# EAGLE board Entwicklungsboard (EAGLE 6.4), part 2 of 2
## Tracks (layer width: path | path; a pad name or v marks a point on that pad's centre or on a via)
1A  (via drill 0.6)
  Top 0.3: v-144.73,27.65 -143.53,26.45 -143.53,24.05 JP15.15
  Bottom 0.3: v-144.73,27.65 -149.73,27.65 -157.63,35.55 IC8.2
1B  (via drill 0.6)
  Top 0.3: v-132.63,35.65 -132.63,46.65 -131.03,48.25 IC9.2
  Bottom 0.3: v-132.63,35.65 -141.63,26.65 -150.43,26.65 -151.43,25.65 -151.43,22.95 -152.53,22.95 JP15.7
1Y
  Top 0.3: IC8.3 -155.03,35.65 -154.53,36.15 -154.53,41.55 -154.03,42.05 -154.03,51.05 -155.03,52.05 MOTOR1.1
1YB
  Top 0.3: IC9.3 -128.33,48.35 -127.13,49.55 -127.13,62.25 -126.43,62.95 -115.73,62.95 -115.73,61.05 MOTOR2.1
2A
  Top 0.3: IC8.7 -144.93,35.55 -145.73,34.75 -145.73,26.25 -146.13,25.85 -146.13,24.15 -144.93,22.95 JP15.13
2B
  Bottom 0.3: IC9.7 -118.33,48.25 -121.03,45.55 -137.83,45.55 -146.03,37.35 -158.13,37.35 -158.73,36.75 -158.73,26.65 -154.63,26.65 -153.93,25.95 -153.93,22.95 -155.03,22.95 JP15.5
2Y
  Top 0.3: IC8.6 -147.53,35.65 -148.93,37.05 -148.93,51.05 -149.93,52.05 MOTOR1.3
2YB
  Top 0.3: IC9.6 -120.73,48.35 -119.73,49.35 -119.73,59.95 -120.73,60.95 MOTOR2.3
3A
  Top 0.3: IC8.10 -144.93,43.15 -146.33,41.75 -146.33,28.25 -148.63,25.95 -148.63,24.05 -147.53,22.95 JP15.11
3B
  Bottom 0.3: IC9.10 -118.33,55.95 -120.63,58.25 -152.23,58.25 -161.93,48.55 -161.93,21.75 -158.73,21.75 -157.63,22.85 JP15.3
3Y
  Top 0.3: IC8.11 -147.43,43.25 -147.43,52.05 MOTOR1.4
3YB
  Top 0.3: IC9.11 -120.83,55.95 -123.33,58.45 -123.33,60.95 MOTOR2.4
4A
  Top 0.3: IC8.15 -157.63,43.15 -156.23,41.75 -156.23,30.75 -151.13,25.65 -151.13,24.05 -150.03,22.95 JP15.9
4B
  Bottom 0.3: IC9.15 -131.03,55.95 -132.73,57.65 -152.03,57.65 -161.33,48.35 -161.33,22.95 -160.23,22.95 JP15.1
4Y
  Top 0.3: IC8.14 -155.13,43.25 -156.33,44.45 -156.33,53.35 -155.63,54.05 -142.43,54.05 -142.43,52.15 MOTOR1.6
4YB
  Top 0.3: IC9.14 -128.43,55.95 -128.43,60.95 MOTOR2.6
+12
  Top 0.3: -45.63,-13.68 S1.3 | -45.63,-9.08 S1.6 -45.53,-10.18 | C2.+ -48.33,2.52 -43.33,-2.48 -39.63,-2.48 TP4.TP -39.53,-2.58 -39.53,-10.08 C3.1 -39.63,-10.18
  Top 0.813: -45.63,-9.08 -45.63,-13.68 | -39.63,-10.18 -45.53,-10.18
  Bottom 0.3: -25.63,-15.18 IC1.1 | -39.43,-10.18 C3.1
  Bottom 0.813: -25.63,-15.18 -30.63,-10.18 -39.43,-10.18
+12V  (via drill 0.6)
  Top 0.3: v-115.83,43.95 -115.73,44.05 -115.73,48.25 IC9.8 | SPI_INPUT.3 -155.53,-10.55 -155.53,3.05 v-153.53,5.05
  Bottom 0.3: -131.63,40.85 -125.93,40.85 -122.83,43.95 v-115.83,43.95 | -131.63,40.85 -137.13,40.85 -142.33,35.65 IC8.8 | v-153.53,5.05 -148.93,9.65 -135.93,9.65 -132.53,13.05 -132.53,34.65 -132.23,34.65 -131.63,35.25 -131.63,40.85
A
  Top 0.3: A1.TP 63.14,149.83 63.14,146.33 10.1 62.79,145.98 62.79,136.18 10.2 62.79,135.83 62.79,130.93 11.1 63.14,130.58 63.14,126.03 66.99,126.03 67.34,125.68 69.79,125.68 70.49,124.98 70.49,123.23 65.59,123.23 63.14,120.78 11.2 62.79,120.78 62.79,115.88 12.1 62.79,115.53 62.79,105.73 12.2 | 18.2 62.79,90.33 62.79,100.13 18.1 62.79,100.48 62.79,105.38 12.2 | TASTATUR1.8 64.89,105.73 63.14,105.73 12.2
B  (via drill 0.6)
  Top 0.3: 59.29,148.43 59.99,147.73 59.99,143.88 56.49,143.88 | 59.29,148.43 58.94,148.78 55.79,148.78 54.74,149.83 B1.TP | 56.49,143.88 54.39,145.98 13.1 | 14.2 54.04,120.78 54.04,130.58 14.1 54.04,130.93 52.99,130.93 v52.29,131.63 | v51.94,133.73 54.04,135.83 13.2 | v56.49,138.98 56.49,143.88 | 19.2 54.04,90.33 54.04,100.13 19.1 54.04,100.48 54.04,103.63 | 54.04,103.63 54.04,105.38 15.2 | 60.34,103.63 60.34,107.13 59.29,108.18 54.39,108.18 54.39,115.53 15.1 | 54.04,103.63 60.34,103.63 | 60.34,103.63 60.34,89.63 61.74,88.23 70.49,88.23 70.49,109.93 68.74,111.68 TASTATUR1.7 68.39,112.03 66.29,112.03 66.29,119.73 67.34,120.78 71.19,120.78 71.19,144.58 64.19,151.58 62.44,151.58 59.29,148.43
  Bottom 0.3: v52.29,131.63 52.29,133.38 v51.94,133.73 51.94,134.43 v56.49,138.98
C  (via drill 0.6)
  Top 0.3: RIGHT1.2 45.29,90.33 45.29,100.13 RIGHT1.1 45.29,100.48 45.29,105.38 17.2 45.29,105.73 45.64,106.08 v47.74,106.08 | C16.TP 45.29,149.83 45.29,146.33 LEFT1.1 44.94,145.98 v44.94,142.13 | 16.2 45.29,118.33 | 45.29,118.33 45.29,115.88 17.1 | 16.2 45.29,130.58 16.1 44.94,130.93 43.89,130.93 v43.19,131.63 | 16.2 | v42.84,133.73 44.94,135.83 LEFT1.2 | v59.64,117.98 59.29,118.33 45.29,118.33
  Bottom 0.3: v43.19,131.63 43.19,133.38 v42.84,133.73 42.84,140.03 v44.94,142.13 | TASTATUR1.6 68.39,114.48 64.89,117.98 v59.64,117.98 v47.74,106.08
CS  (via drill 0.6)
  Top 0.3: IC2.11 -134.83,17.55 -134.83,19.45 -139.23,19.45 -139.93,18.75 -139.93,18.15 -146.93,11.15 -146.93,7.25 -147.43,6.75 IC3.11 -147.53,6.65 -147.53,5.55 v-148.03,5.05
  Bottom 0.3: SPI_INPUT.8 -156.93,0.75 -153.63,0.75 -151.03,3.35 -151.03,5.05 v-148.03,5.05
D
  Top 0.3: 36.19,128.83 36.19,130.58 F1.1 | 36.19,128.83 36.19,120.78 F1.2 | 29.19,133.38 33.74,133.38 36.19,135.83 CANCEL1.2 | 29.19,133.38 27.09,131.28 27.09,128.83 | 36.19,128.83 27.09,128.83 | 36.19,98.38 36.19,100.13 ENTER1.1 | 36.19,98.38 36.19,90.33 ENTER1.2 | 28.84,102.58 27.09,100.83 27.09,98.38 36.19,98.38 | 28.84,102.58 29.19,102.93 33.74,102.93 36.19,105.38 F3.2 | 28.84,108.18 36.19,115.53 F3.1 | 28.84,102.58 28.84,108.18 | 27.09,128.83 27.09,108.18 28.84,108.18 | 36.54,148.08 36.54,146.33 CANCEL1.1 | 36.54,148.08 36.54,149.83 D3.TP 36.89,150.18 38.99,152.28 66.99,152.28 69.79,149.48 73.24,145.67 73.24,120.78 72.89,120.43 72.24,120.43 68.74,116.93 TASTATUR1.5 | 29.19,133.38 29.19,144.23 28.49,144.23 27.09,145.63 27.09,148.08 36.54,148.08
DATA+
  Top 0.3: R52.1 59.36,-15.02 59.36,-12.62 64.16,-12.62 X1.3
DATA-  (via drill 0.6)
  Top 0.3: v60.86,-10.82 59.96,-10.82 59.36,-10.22 R53.1 | v61.76,-13.82 62.06,-13.52 64.16,-13.52 X1.2
  Bottom 0.3: v60.86,-10.82 61.76,-11.72 v61.76,-13.82
E  (via drill 0.6)
  Top 0.3: E1.TP 29.19,145.98 31.64,145.98 CANCEL1.3 31.99,145.98 34.09,143.88 40.74,143.88 | 40.74,143.88 40.74,145.98 LEFT1.3 | 40.74,143.88 40.74,141.08 | 40.74,141.08 40.74,137.93 | 40.74,137.93 40.74,136.18 LEFT1.4 | 40.74,137.93 33.74,137.93 31.99,136.18 CANCEL1.4 | 10.3 58.24,146.33 56.49,148.08 51.59,148.08 49.84,146.33 13.3 49.49,145.98 49.49,141.08 | v62.09,125.68 62.09,128.83 61.74,128.83 59.99,130.58 59.99,135.83 58.59,135.83 10.4 58.24,136.18 56.49,137.93 51.59,137.93 49.84,136.18 13.4 49.49,136.18 49.49,141.08 | 49.49,141.08 40.74,141.08
  Bottom 0.3: v62.09,125.68 62.09,119.73 68.39,119.73 TASTATUR1.4
F  (via drill 0.6)
  Top 0.3: 58.59,124.63 58.59,130.58 11.3 58.24,130.93 56.49,132.68 47.74,132.68 | 58.59,124.63 58.59,120.78 11.4 | v64.89,124.98 64.54,124.63 58.59,124.63 | 14.4 49.49,120.78 49.49,130.58 14.3 49.49,130.93 47.74,132.68 | F2.TP 29.19,130.93 31.64,130.93 F1.3 31.99,130.93 33.74,132.68 38.99,132.68 | 40.74,120.78 40.74,130.58 16.3 40.74,130.93 38.99,132.68 | 40.74,120.78 38.64,118.68 34.09,118.68 31.99,120.78 F1.4 | 40.74,120.78 16.4 | 38.99,132.68 47.74,132.68
  Bottom 0.3: v64.89,124.98 64.89,122.18 68.39,122.18 TASTATUR1.3
G
  Top 0.3: TASTATUR1.2 68.39,124.28 68.04,123.93 63.14,123.93 60.69,121.48 60.69,115.88 58.59,115.88 12.3 58.24,115.88 56.49,117.63 51.59,117.63 49.84,115.88 15.3 49.49,115.53 47.39,113.43 40.74,113.43 | 12.4 58.24,105.73 56.49,107.48 51.59,107.48 49.84,105.73 15.4 49.49,105.73 47.74,107.48 40.74,107.48 | G1.TP 29.19,115.53 31.64,115.53 F3.3 31.99,115.88 33.74,117.63 38.99,117.63 40.74,115.88 17.3 40.74,115.53 40.74,113.43 | 40.74,113.43 40.74,107.48 | 40.74,107.48 40.74,105.73 17.4 | 40.74,107.48 33.74,107.48 31.99,105.73 F3.4
GND
  Top 0.8: C5.1 -8.63,39.42 -8.13,38.92 -8.13,36.12 -6.93,34.92 -6.93,21.22 -9.03,19.12 SG1.- | -0.33,38.02 -1.63,38.02 -1.63,48.52 U1.12 -2.83,49.92 -6.53,53.62 -6.53,63.62 -7.73,64.82 U1.31 | -0.33,38.02 2.37,38.02 2.77,38.42 2.77,38.92 3.27,39.42 C6.2 | -0.33,38.02 -0.33,32.12 0.67,32.12 7.27,25.52 11.27,25.52 JP3.3 11.67,25.32 20.47,16.52 20.47,4.32 19.07,2.92 IR1.GND 18.87,2.52 13.57,-2.78 13.57,-15.08 11.37,-17.28 C8.- 11.27,-17.68 -2.63,-17.68 C7.2 | JP19.2 20.17,85.22 19.07,86.32 19.07,86.52 -3.13,108.72 -7.43,108.72 R22.2 -7.83,109.02 -10.53,109.02 -10.93,109.42 -21.43,109.42 -21.43,109.22 R23.2 -21.83,108.92 -31.83,108.92 R20.2 -32.23,108.72 -35.13,108.72 -35.13,81.72 R10.2 -35.43,81.42 -38.23,81.42 | C9.- -49.23,41.92 -49.23,34.82 -50.93,33.12 C1.- -50.83,32.72 -49.73,31.62 -49.73,19.22 -48.63,18.12 C10.1 -48.43,17.82 -48.43,10.22 C2.- -48.13,9.92 -37.53,-0.68 -37.53,-15.78 -39.43,-17.68 C3.2 | ICSP.3 -40.73,58.52 -39.63,58.52 -39.63,59.32 -38.33,60.62 -38.33,73.62 C4.- -38.23,74.02 -38.23,81.42 | -50.93,83.82 -50.93,83.62 S2.4 | -38.23,81.42 -40.83,81.42 -40.83,83.52 S2.3 -41.23,83.62 -50.53,83.62 S2.4 | TP6.TP -52.13,87.62 -51.13,86.62 -51.13,84.12 S2.4
  Bottom 0.8: SG1.- -9.03,19.12 -2.73,25.42 11.27,25.42 JP3.3 | GND.1 -43.33,-20.18 -41.93,-20.18 -39.53,-17.78 C3.2 -39.33,-17.38 -23.03,-17.38 | -23.03,-17.38 -23.03,-15.28 IC1.2 | -23.03,-17.38 -22.73,-17.58 -22.63,-17.68 -2.73,-17.68 C7.2 | C9.- -49.13,42.02 -46.63,44.52 -46.63,58.42 -40.83,58.42 ICSP.3
GNDCOM
  Top 0.3: 47.91,20.93 47.91,27.93 C15.1 | 46.76,20.93 45.11,20.93 44.41,20.23 | 46.76,20.93 47.91,20.93 | 62.36,-11.12 61.46,-12.02 48.86,-12.02 43.16,-17.72 JP16.1 | 62.66,-11.12 64.16,-11.12 X1.5 62.66,-11.12 | 62.66,-11.12 62.36,-11.12 | 46.76,20.98 46.76,20.93 | 49.26,15.68 47.26,13.68 45.86,13.68 45.86,2.48 IC10.7 | 49.26,15.68 49.26,20.98 47.96,20.98 47.91,20.93 | IC10.26 48.46,-4.82 47.86,-4.82 IC10.25 47.86,-4.92 47.86,-6.02 | 45.06,-5.92 45.26,-5.72 45.26,-4.92 IC10.21 | 45.06,-5.92 44.96,-6.02 43.26,-6.02 43.26,-4.92 IC10.18 | 47.86,-6.02 45.16,-6.02 45.06,-5.92 | 58.56,-5.82 59.26,-5.12 C11.2 59.26,-5.02 60.56,-3.72 67.06,-3.72 67.16,-3.62 67.16,8.08 66.16,9.08 55.86,9.08 49.26,15.68 | 58.56,-5.82 58.16,-6.22 48.06,-6.22 47.86,-6.02 | 58.56,-5.82 62.16,-9.42 62.26,-9.42 62.26,-11.02 62.36,-11.12
  Bottom 0.3: IC11.15 48.26,46.83 53.16,41.93 53.16,36.33 54.21,35.28 X2.5 54.21,34.93 54.21,34.23 48.26,28.28 C15.1 48.26,27.93 49.31,26.88
  pour Bottom (isolate 0.406): 74.78,61.01 74.78,-22.81 30.33,-22.81 30.33,61.01
GNDI2C
  Top 0.3: -154.02,130.4 -154.02,128.65 -153.32,127.95 -153.32,127.25 U$1.4 | -154.02,130.4 -154.02,131.8 -154.37,132.15 U$1.6 | -154.02,130.4 -162.42,130.4 -162.42,143.35 R65.E
  pour Bottom (isolate 0.406): -172.87,153.72 -80.16,153.72 -80.16,80.06 -172.87,80.06
GNDSPI  (via drill 0.6)
  Top 0.3: LED17.13 -106.83,-1.05 | -106.83,-1.05 LED17.14 -106.93,-2.45 -114.83,-2.45 -114.83,-10.85 -117.73,-13.75 -117.73,-14.35 -118.73,-15.35 -127.13,-15.35 -127.13,-16.35 IC5.8 -127.23,-16.55 -129.93,-19.25 -156.33,-19.25 -156.33,-13.95 SPI_INPUT.2 -156.23,-13.85 -154.93,-12.55 -154.93,-6.95 -149.03,-1.05 -149.03,6.25 -148.73,6.55 IC3.10 -148.73,6.75 -148.23,7.25 -148.23,12.15 -146.23,14.15 -146.23,16.25 IC3.17 -146.13,16.25 IC3.16 -144.83,16.25 -143.73,16.25 IC3.15 -143.63,16.35 -143.63,20.05 -141.23,20.05 | -92.73,-1.05 -92.73,6.45 -91.63,7.55 LED17.9 | -92.73,-1.05 -92.73,-3.95 -91.63,-5.05 LED17.4 | -92.73,-1.05 -106.83,-1.05 | LED18.13 LED18.14 | IC4.8 -71.33,3.95 -78.83,11.45 -78.83,19.05 IC7.8 | LED18.4 -92.73,23.95 -92.73,34.35 -91.63,35.45 LED18.9 | IC8.13 -152.53,43.25 -150.03,43.25 IC8.12 | MOTOR1.2 -152.53,52.05 -152.53,43.35 IC8.13 | IC8.4 -152.53,35.65 -152.53,43.15 IC8.13 | -124.63,48.35 -123.43,48.35 IC9.5 -123.23,48.25 -123.23,45.75 -119.53,42.05 IC6.8 | -124.63,48.35 -125.83,48.35 IC9.4 | -124.63,55.95 -123.43,55.95 IC9.12 | -124.63,55.95 -125.83,55.95 IC9.13 -125.83,56.05 -125.83,60.95 MOTOR2.5 | -124.63,55.95 -124.63,48.35 | -141.23,20.05 -134.63,20.05 -134.03,19.45 -134.03,18.05 -133.53,17.55 IC2.10 | v-142.03,27.65 -141.23,26.85 -141.23,20.05
  Bottom 0.3: -88.63,19.85 -79.63,19.85 -78.93,19.15 IC7.8 | -88.63,19.85 LED18.4 -91.73,22.85 -94.03,25.15 -106.43,25.15 LED18.14 | LED17.9 -91.53,7.65 -88.73,10.45 -88.73,19.75 -88.63,19.85 | IC8.4 -152.53,35.65 -150.03,35.65 IC8.5 -149.93,35.55 v-142.03,27.65 | MOTOR1.2 -152.53,52.15 -150.63,54.05 -146.83,54.05 -144.93,52.15 MOTOR1.5 -144.83,52.05 -142.83,50.05 -127.63,50.05 -125.93,48.35 IC9.4 | MOTOR2.2 -118.33,61.05 -120.23,62.95 -123.93,62.95 -125.83,61.05 MOTOR2.5
H  (via drill 0.6)
  Top 0.3: 19.4 49.49,90.33 49.49,100.13 19.3 | H1.TP 29.19,100.48 31.64,100.48 ENTER1.3 31.99,100.48 33.74,102.23 38.99,102.23 40.74,100.48 RIGHT1.3 40.74,100.13 40.74,90.33 RIGHT1.4 40.74,89.98 38.99,88.23 | 38.99,88.23 33.74,88.23 31.99,89.98 ENTER1.4 | 38.99,88.23 47.74,88.23 49.49,89.98 19.4 | 18.3 58.59,100.13 58.59,90.33 18.4 58.59,89.98 60.34,88.23 | v72.59,119.38 72.24,110.54 72.24,88.45 71.32,87.53 61.04,87.53 60.34,88.23 | 60.34,88.23 51.59,88.23 49.84,89.98 19.4
  Bottom 0.3: v72.59,119.38 72.59,122.88 68.74,126.73 TASTATUR1.1
MCLR
  Top 0.3: D2.C -44.53,49.62 -40.83,53.32 ICSP.1
  Bottom 0.3: U1.1 -30.63,49.62 -34.33,53.32 -40.73,53.32 ICSP.1
N$1
  Top 0.3: C5.2 -6.73,39.42 -4.03,42.12 -4.03,44.42 Q1.1
  Bottom 0.3: U1.13 -0.23,49.52 -3.93,45.82 -3.93,44.52 Q1.1
N$2
  Top 0.3: R2.1 -20.43,138.72 -20.43,134.72 JP5.8
N$3
  Top 0.3: C6.1 1.37,39.42 1.17,39.62 1.17,44.42 Q1.2 1.17,44.62 1.17,48.32 2.37,49.52 U1.14
N$4
  Top 0.3: JP5.7 R3.1
N$5
  Top 0.3: R13.1 -42.33,113.12 -38.33,113.12 JP10.8
N$6
  Top 0.3: JP10.7 R14.1
N$7
  Top 0.3: R15.1 -42.33,118.22 -38.33,118.22 JP10.6
N$8
  Top 0.3: R16.1 -42.33,120.72 -38.33,120.72 JP10.5
N$9
  Top 0.3: R17.1 -42.33,123.32 -38.33,123.32 JP10.4
N$10
  Top 0.3: R18.1 -42.33,125.82 -38.33,125.82 JP10.3
N$11
  Top 0.3: JP10.2 R19.1
N$12
  Top 0.3: R21.1 -42.33,130.92 -38.33,130.92 JP10.1
N$13
  Top 0.3: R13.2 -44.33,113.02 -47.93,109.42 -47.93,97.02 -49.63,95.32 LED9.K
N$14
  Top 0.3: R15.2 -44.33,118.12 -49.63,112.82 -49.63,110.62 LED11.K
N$15
  Top 0.3: R16.2 -44.33,120.62 -49.63,120.62 -49.63,118.22 LED12.K
N$16
  Top 0.3: R17.2 -44.33,123.32 -49.63,123.32 -49.63,125.72 LED13.K
N$17
  Top 0.3: R21.2 -44.33,130.92 -47.93,134.52 -47.93,146.92 -49.63,148.62 LED16.K
N$18
  Top 0.3: R18.2 -44.33,125.82 -49.63,131.12 -49.63,133.32 LED14.K
N$19
  Top 0.3: R14.2 -44.33,115.62 -48.53,111.42 -48.53,104.02 -49.63,102.92 LED10.K
N$20
  Top 0.3: R19.2 -44.33,128.32 -48.53,132.52 -48.53,139.92 -49.63,141.02 LED15.K
N$21
  Top 0.3: R4.1 -15.33,138.72 -15.33,134.72 JP5.6
N$22
  Top 0.3: R6.1 -12.83,138.72 -12.83,134.72 JP5.5
N$23
  Top 0.3: R7.1 -10.23,138.72 -10.23,134.72 JP5.4
N$24
  Top 0.3: R9.1 -7.73,138.72 -7.73,134.72 JP5.3
N$25
  Top 0.3: JP5.2 R11.1
N$26
  Top 0.3: R12.1 -2.63,138.72 -2.63,134.72 JP5.1
N$27
  Top 0.3: R2.2 -20.53,140.72 -27.33,147.52 -38.23,147.52 -38.23,148.62 LED1.K
N$28
  Top 0.3: R4.2 -15.43,140.72 -22.93,148.22 -22.93,148.62 LED3.K
N$29
  Top 0.3: R6.2 -12.93,140.72 -15.33,143.12 -15.33,148.62 LED4.K
N$30
  Top 0.3: R7.2 -10.23,140.72 -7.83,143.12 -7.83,148.62 LED5.K
N$31
  Top 0.3: R12.2 -2.63,140.72 4.17,147.52 15.07,147.52 15.07,148.62 LED8.K
N$32
  Top 0.3: R3.2 -17.93,140.72 -25.83,148.62 -30.63,148.62 LED2.K
N$33
  Top 0.3: R9.2 -7.73,140.72 -0.23,148.22 -0.23,148.62 LED6.K
N$34
  Top 0.3: R11.2 -5.23,140.72 2.67,148.62 7.47,148.62 LED7.K
N$35
  Top 0.3: IC11.14 47.91,44.38 46.16,42.63 46.16,40.88 54.21,40.88 X2.3
N$36
  Top 0.3: IC11.13 48.26,42.28 49.31,43.33 54.21,43.33 X2.2
N$37
  Bottom 0.3: IC11.2 40.56,47.18 42.31,48.93 42.31,51.38 40.56,53.13 C14.2
N$38
  Bottom 0.3: IC11.6 40.56,36.68 42.31,34.93 42.31,30.03 40.56,28.28 C15.2
N$39
  Top 0.3: IC11.3 40.21,44.73 38.11,46.83 34.26,46.83 C12.2
N$40
  Top 0.3: IC11.1 40.21,49.63 35.31,54.53 34.26,54.53 C12.1
N$41
  Top 0.3: IC11.4 40.21,42.28 39.51,42.98 34.26,42.98 C13.1
N$42
  Top 0.3: IC11.5 40.21,39.13 36.71,35.63 34.26,35.63 C13.2
N$43  (via drill 0.6)
  Top 0.3: v47.46,-2.22 45.86,-2.22 45.86,-4.82 IC10.22 | v55.16,5.48 57.26,7.58 R56.1
  Bottom 0.3: v55.16,5.48 v47.46,-2.22
N$44  (via drill 0.6)
  Top 0.3: v51.96,-0.62 49.36,-3.22 46.56,-3.22 46.56,-4.82 IC10.23 | v56.16,12.58 56.16,13.98 57.26,13.98 R55.1
  Bottom 0.3: v51.96,-0.62 56.16,3.58 v56.16,12.58
N$45
  Top 0.3: 59.36,17.68 LED19.K 59.26,17.58 59.26,14.08 R55.2
N$46
  Top 0.3: 63.26,7.48 LED20.K 63.16,7.58 59.26,7.58 R56.2
N$47
  Top 0.3: IC10.17 42.66,-4.82 42.66,-3.22 34.46,-3.22 34.16,-2.92 34.16,0.78 47.46,0.78 47.86,0.38 53.06,0.38 57.26,-3.82 57.26,-5.02 C11.1
N$48
  Top 0.3: R22.1 -7.83,107.02 -8.03,106.82 -8.03,104.12 INT1.4 -8.03,104.02 -8.03,94.12 INT1.3
N$49
  Top 0.3: R52.2 57.26,-15.32 52.76,-19.82 41.36,-19.82 41.36,-4.92 IC10.15
N$50
  Top 0.3: IC12.4 -97.67,127.25 -93.47,127.25 -93.47,128.65 -91.37,130.75 -82.27,130.75 -82.27,104.5 -85.07,101.7 KEYBOARD.1
N$51
  Top 0.3: IC12.5 -98.02,124.45 -110.62,111.85 -113.77,111.85 -113.77,107.65 -112.72,106.6 -87.17,106.6 -87.17,106.25 -85.42,104.5 KEYBOARD.2
N$52  (via drill 0.6)
  Top 0.3: 43.71,29.33 48.61,29.33 50.36,27.58 50.36,19.18 JP18.3 | v49.86,13.68 49.86,2.48 IC10.1
  Bottom 0.3: 50.36,18.88 JP18.3 50.26,18.78 50.26,14.08 v49.86,13.68
N$53  (via drill 0.6)
  Top 0.3: v-94.52,122 -92.07,119.55 -92.07,113.6 -85.42,106.95 KEYBOARD.3
  Bottom 0.3: v-94.52,122 -97.67,122 IC12.6
N$54
  Bottom 0.3: IC12.7 -97.67,119.2 -96.62,119.2 -87.17,109.75 -86.82,109.75 -86.47,109.4 -85.42,109.4 KEYBOARD.4
N$55
  Top 0.3: R53.2 57.26,-9.92 41.96,-9.92 41.96,-4.92 IC10.16
N$56
  Bottom 0.3: IC11.11 45.81,34.58 45.81,19.18 JP18.1
N$57
  Top 0.3: JP6.1 R8.2
N$58  (via drill 0.6)
  Top 0.3: v47.16,12.68 47.16,2.48 IC10.5 | v46.86,14.68 42.46,19.08 41.76,19.08 JP17.3
  Bottom 0.3: 43.76,17.08 41.76,19.08 JP17.3 | v47.16,12.68 46.86,12.98 v46.86,14.68
N$59
  Top 0.3: IC11.12 47.91,39.13 41.96,33.18 36.86,33.18 | 36.86,33.18 36.71,33.18 | 36.86,33.18 36.86,19.18 JP17.1 | 36.86,33.28 36.86,33.18
N$60
  Top 0.3: IC12.9 -90.32,116.75 -85.42,111.85 KEYBOARD.5
N$61
  Top 0.3: IC12.10 -90.32,119.2 -85.42,114.3 KEYBOARD.6
N$62
  Top 0.3: IC12.11 -90.32,121.65 -82.97,121.65 -82.97,119.2 -85.07,117.1 KEYBOARD.7
N$63
  Top 0.3: IC12.12 -90.32,124.45 -92.07,122.7 -92.07,121.3 -91.37,120.6 -85.42,120.6 -85.42,119.55 KEYBOARD.8
N$64
  Top 0.3: IC10.19 43.96,-4.82 43.96,-2.22 35.46,-2.22 R54.2
N$65
  Bottom 0.3: IC4.7 -71.23,1.25 -68.93,-1.05 -68.93,-19.25 -146.33,-19.25 -148.83,-16.75 -148.83,-13.95 -149.93,-13.95 JP13.15
N$66
  Top 0.3: R5.2 -28.03,70.92 -28.03,85.12 JP6.2
N$67
  Bottom 0.3: IC4.1 -71.33,-13.95 -72.43,-15.05 -146.33,-15.05 -147.43,-13.95 JP13.13
N$68  (via drill 0.6)
  Top 0.3: v-143.73,-18.25 -143.73,-15.15 -144.93,-13.95 JP13.11
  Bottom 0.3: v-143.73,-18.25 -69.53,-18.25 -69.53,-13.15 -71.23,-11.45 IC4.2
N$69  (via drill 0.6)
  Top 0.3: v-81.33,-10.85 -81.33,-7.75 -77.83,-7.75 -71.33,-1.25 IC4.6
  Bottom 0.3: v-81.33,-10.85 -81.83,-11.35 -117.33,-11.35 -118.43,-10.25 -137.53,-10.25 -140.03,-12.75 -141.23,-12.75 -142.33,-13.85 JP13.9
N$70
  Bottom 0.3: IC5.7 -127.23,-13.85 -128.33,-12.75 -138.73,-12.75 -139.83,-13.85 JP13.7
N$71  (via drill 0.6)
  Top 0.3: v-136.83,-2.75 -137.23,-3.15 -137.23,-13.85 JP13.5
  Bottom 0.3: v-136.83,-2.75 -135.83,-1.75 -130.23,-1.75 -127.23,1.25 IC5.1
N$72  (via drill 0.6)
  Top 0.3: v-132.23,-2.75 -133.83,-4.35 -133.83,-9.15 -134.73,-10.05 -134.73,-13.85 JP13.3
  Bottom 0.3: v-132.23,-2.75 -128.73,-2.75 -127.23,-1.25 IC5.2
N$73  (via drill 0.6)
  Top 0.3: v-130.73,-11.75 -132.23,-13.25 JP13.1
  Bottom 0.3: v-130.73,-11.75 -127.53,-11.75 -127.23,-11.45 IC5.6
N$74  (via drill 0.6)
  Top 0.3: v-134.83,-4.75 -134.83,-3.95 -130.93,-0.05 -130.93,7.95 IC2.21 | v-145.63,-10.45 -148.83,-13.65 -148.83,-15.35 -149.93,-16.45 JP13.16
  Bottom 0.3: v-134.83,-4.75 -140.53,-10.45 v-145.63,-10.45
N$75  (via drill 0.6)
  Top 0.3: v-132.83,-4.75 -130.23,-2.15 -130.23,7.45 -129.73,7.95 IC2.22 | v-144.03,-11.45 -146.33,-13.75 -146.33,-15.35 -147.43,-16.45 JP13.14
  Bottom 0.3: v-132.83,-4.75 -139.53,-11.45 v-144.03,-11.45
N$76
  Top 0.3: R25.2 -87.53,-10.15 -91.53,-10.15 LED17.2
N$77  (via drill 0.6)
  Top 0.3: v-112.03,-3.45 -112.03,-4.15 -112.83,-4.95 R24.1
  Bottom 0.3: v-112.03,-3.45 -111.73,-3.75 -78.93,-3.75 IC4.12
N$78  (via drill 0.6)
  Top 0.3: v-90.33,-6.25 -111.63,-6.25 -112.03,-6.65 -112.03,-6.75 -112.83,-7.55 R37.1
  Bottom 0.3: v-90.33,-6.25 -78.93,-6.25 IC4.13
N$79  (via drill 0.6)
  Top 0.3: v-84.23,-8.85 -84.23,-10.05 -85.53,-10.05 R25.1 | v-82.23,-7.25 -80.63,-5.65 -80.63,-0.45 -78.93,1.25 IC4.10
  Bottom 0.3: v-84.23,-8.85 -82.63,-7.25 v-82.23,-7.25
N$80
  Top 0.3: R38.1 -85.53,-7.55 -83.83,-5.85 -83.83,1.15 -80.03,4.95 -77.13,4.95 -77.13,0.55 -78.83,-1.15 IC4.11
N$81
  Top 0.3: R39.1 -85.53,-12.65 -83.23,-10.35 -83.23,-0.45 -78.93,3.85 IC4.9
N$82
  Top 0.3: R26.1 -112.83,-12.65 -112.03,-13.45 -112.03,-13.55 -108.23,-17.35 -80.63,-17.35 -80.63,-13.15 -78.93,-11.45 IC4.15
N$83  (via drill 0.6)
  Top 0.3: v-107.73,-8.95 -111.83,-8.95 -112.03,-9.15 -112.03,-9.25 -112.83,-10.05 R40.1
  Bottom 0.3: v-107.73,-8.95 -107.63,-9.05 -85.43,-9.05 -84.63,-9.85 -79.93,-9.85 -78.93,-8.85 IC4.14
N$84  (via drill 0.6)
  Top 0.3: v-115.83,-2.55 -115.83,2.15 -112.93,5.05 R41.1
  Bottom 0.3: v-115.83,-2.55 -119.53,-6.25 IC5.13
N$85
  Top 0.3: R27.1 -112.93,7.65 -116.83,3.75 -116.83,-10.85 -118.43,-12.45 -121.33,-12.45 -121.33,-10.65 IC5.12
N$86
  Top 0.3: R42.1 -85.63,5.15 -86.33,5.85 -86.33,6.05 -89.23,8.95 -117.73,8.95 -117.73,-9.55 -119.53,-11.35 IC5.11
N$87  (via drill 0.6)
  Top 0.3: v-84.83,-4.75 -84.43,-4.35 -84.43,-1.05 -85.53,0.05 R28.1
  Bottom 0.3: v-84.83,-4.75 -84.43,-5.15 -77.83,-5.15 -77.13,-5.85 -77.13,-12.65 -89.83,-12.65 -91.13,-13.95 -119.53,-13.95 IC5.10
N$88
  Top 0.3: R43.1 -85.63,-2.55 -86.33,-3.25 -86.33,-3.65 -90.43,-7.75 -90.43,-8.15 -91.33,-9.05 -105.63,-9.05 -105.63,-10.65 -106.43,-11.45 -114.63,-11.45 -114.63,-12.05 -119.03,-16.45 IC5.9
N$89  (via drill 0.6)
  Top 0.3: v-114.83,0.65 -112.93,2.55 R29.1
  Bottom 0.3: v-114.83,0.65 -116.63,-1.15 -119.53,-1.15 IC5.15
N$90  (via drill 0.6)
  Top 0.3: v-84.03,2.55 -85.53,2.55 R44.1
  Bottom 0.3: v-84.03,2.55 -87.83,-1.25 -115.93,-1.25 -118.43,-3.75 IC5.14
N$91
  Top 0.3: R37.2 -110.93,-7.65 -106.83,-7.65 LED17.16
N$92
  Top 0.3: R24.2 -110.93,-5.05 -106.83,-5.05 LED17.15
N$93  (via drill 0.6)
  Top 0.3: v-88.93,-7.65 -87.53,-7.65 R38.2
  Bottom 0.3: v-88.93,-7.65 -91.53,-7.65 LED17.3
N$94
  Top 0.3: R39.2 -91.53,-12.65 -91.53,-12.75 LED17.1
N$95
  Top 0.3: R26.2 -106.83,-12.65 LED17.18
N$96
  Top 0.3: R40.2 -110.93,-10.15 -106.83,-10.15 LED17.17
N$97
  Top 0.3: R41.2 -110.93,5.15 -106.83,5.15 LED17.11
N$98
  Top 0.3: R27.2 -110.93,7.75 -106.83,7.75 LED17.10
N$99
  Top 0.3: R42.2 -87.53,5.05 -91.53,5.05 LED17.8
N$100
  Top 0.3: R28.2 -91.53,0.05 -91.53,-0.05 LED17.6
N$101
  Top 0.3: R43.2 -87.53,-2.55 -91.53,-2.55 LED17.5
N$102
  Top 0.3: R29.2 -110.93,2.65 -106.83,2.65 LED17.12
N$103
  Top 0.3: R44.2 -87.53,2.55 -91.53,2.55 LED17.7
N$104  (via drill 0.6)
  Top 0.3: v-130.63,-16.45 -130.63,-13.05 -128.93,-11.35 -128.93,7.45 -128.43,7.95 IC2.23
  Bottom 0.3: v-130.63,-16.45 -131.83,-17.65 -142.93,-17.65 -144.03,-16.55 -144.93,-16.55 JP13.12
N$105  (via drill 0.6)
  Top 0.3: v-127.63,6.25 -127.63,7.55 -127.23,7.95 IC2.24 | v-131.93,5.25 -141.23,-4.05 -141.23,-15.35 -142.33,-16.45 JP13.10
  Bottom 0.3: v-127.63,6.25 -128.63,5.25 v-131.93,5.25
N$106  (via drill 0.6)
  Top 0.3: v-126.03,6.25 -126.03,7.85 -125.93,7.95 IC2.25 | v-131.93,3.85 -138.73,-2.95 -138.73,-15.35 -139.83,-16.45 JP13.8
  Bottom 0.3: v-126.03,6.25 -128.43,3.85 v-131.93,3.85
N$107  (via drill 0.6)
  Top 0.3: IC2.26 -124.83,7.75 v-124.83,4.65 | v-131.93,2.45 -135.83,-1.45 -135.83,-13.35 -136.13,-13.65 -136.13,-15.35 -137.23,-16.45 JP13.6
  Bottom 0.3: v-124.83,4.65 -127.03,2.45 v-131.93,2.45
N$108  (via drill 0.6)
  Top 0.3: v-123.83,-5.15 -123.83,7.55 -123.43,7.95 IC2.27 | v-131.63,-7.75 -133.63,-9.75 -133.63,-15.35 -134.73,-16.45 JP13.4
  Bottom 0.3: v-123.83,-5.15 -126.43,-7.75 v-131.63,-7.75
N$109
  Top 0.3: JP13.2 -132.23,-17.45 -130.23,-17.45 -129.63,-16.85 -129.63,-12.85 -126.43,-12.85 -122.53,-8.95 -122.53,7.55 -122.13,7.95 IC2.28
N$110  (via drill 0.6)
  Top 0.3: v-116.83,49.95 -116.83,47.55 -117.83,46.55 -117.83,45.55 -117.73,45.45 -117.73,41.25 -119.53,39.45 IC6.7
  Bottom 0.3: v-116.83,49.95 -110.93,55.85 -108.13,55.85 JP14.15
N$111  (via drill 0.6)
  Top 0.3: v-114.73,24.45 -113.73,25.45 -113.73,29.35 -113.93,29.55 -113.93,45.95 -106.73,53.15 -106.73,54.75 -105.63,55.85 JP14.13
  Bottom 0.3: v-114.73,24.45 -119.33,24.45 -119.53,24.25 IC6.1
N$112  (via drill 0.6)
  Top 0.3: v-114.73,27.05 -114.73,47.05 -110.63,51.15 -110.63,55.85 -108.83,57.65 -103.03,57.65 -103.03,55.95 JP14.11
  Bottom 0.3: v-114.73,27.05 -119.23,27.05 -119.53,26.75 IC6.2
N$113  (via drill 0.6)
  Top 0.3: v-103.83,43.95 -101.63,46.15 -101.63,54.75 -100.53,55.85 JP14.9
  Bottom 0.3: v-103.83,43.95 -112.53,43.95 -119.53,36.95 IC6.6
N$114
  Top 0.3: IC7.7 -78.93,21.65 -82.63,25.35 -82.63,44.05 -91.73,53.15 -91.73,53.85 -92.63,54.75 -97.93,54.75 -97.93,55.85 JP14.7
N$115
  Bottom 0.3: IC7.1 -78.93,36.95 -89.13,47.15 -89.13,54.75 -94.23,54.75 -95.33,55.85 JP14.5
N$116
  Top 0.3: IC7.2 -78.93,34.35 -81.43,36.85 -81.43,48.65 -89.83,57.05 -92.83,57.05 -92.83,55.95 JP14.3
N$117
  Top 0.3: IC7.6 -78.93,24.25 -82.03,27.35 -82.03,47.65 -90.23,55.85 JP14.1
N$118
  Top 0.3: R20.1 -31.83,107.02 -31.63,106.82 -31.63,104.12 INT2.3 -31.53,104.02 -31.53,94.12 INT2.4
N$119
  pour Bottom (isolate 0.61): 26.52,83.87 26.52,153.72 76.05,153.72 76.05,83.87
N$120
  pour Top (isolate 0.813): -56.03,154.99 22.71,154.99 22.71,-22.81 -56.03,-22.81
N$121
  Bottom 0.305: 43.93,0.34 43.98,0.39
N$122
  Top 0.3: JP2.1 -9.03,31.72 SG1.+
N$137
  Top 0.3: JP3.2 18.87,15.32 18.87,10.22 IR1.VO
N$150  (via drill 0.6)
  Top 0.3: v-150.83,17.95 -150.83,16.75 -151.23,16.35 IC3.21
  Bottom 0.3: v-150.83,17.95 -146.13,22.65 -146.13,24.25 -143.63,24.25 -142.43,25.45 JP15.16
N$151
  Top 0.3: JP15.14 -144.93,24.65 -143.73,23.45 -143.73,21.15 -149.03,21.15 -152.03,18.15 -152.03,16.85 -152.53,16.35 IC3.22
N$152  (via drill 0.6)
  Top 0.3: IC3.23 -153.33,16.75 v-153.33,17.95
  Bottom 0.3: v-153.33,17.95 -148.63,22.65 -148.63,25.45 JP15.12
N$153
  Top 0.3: IC3.24 -155.03,16.35 -154.63,16.75 -154.63,18.25 -151.13,21.75 -148.83,21.75 -148.83,23.45 -149.93,24.55 -149.93,25.45 JP15.10
N$154
  Top 0.3: IC3.25 -156.33,16.35 -155.83,16.85 -155.83,20.55 -153.73,22.65 -153.73,24.35 -152.63,25.45 JP15.8
N$155
  Top 0.3: IC3.26 -157.63,16.35 -157.13,16.85 -157.13,21.75 -156.23,22.65 -156.23,24.35 -155.13,25.45 JP15.6
N$156
  Top 0.3: JP15.4 -158.83,24.25 -158.83,16.35 IC3.27
N$157
  Top 0.3: IC3.28 -160.23,16.35 -161.33,17.45 -161.33,24.35 -160.23,25.45 JP15.2
N$160
  Top 0.3: R23.1 -21.73,107.02 -21.53,106.82 -21.53,104.12 INT3.3 -21.43,104.02 -21.43,94.12 INT3.4
N$162
  Top 0.3: R57.1 -152.27,93.65 -146.32,87.7 -146.32,87.35 -145.27,86.3 -123.57,86.3 -123.57,96.1 -120.42,99.25 -117.62,99.25 -117.62,106.25 -119.37,108 IC13.4
N$163
  Top 0.3: -49.63,-20.18 +12V1.1 | -49.63,-13.78 S1.2 -49.63,-13.68 | -49.63,-9.08 S1.5
  Top 0.813: -49.63,-13.78 -49.63,-20.18 | -49.63,-13.68 -49.63,-9.08
N$164
  Top 0.3: R61.1 -144.92,94 -135.47,103.45 -121.47,103.45 -119.72,105.2 IC13.5
N$166
  Top 0.3: R46.2 -87.53,17.75 -91.53,17.75 LED18.2
N$167  (via drill 0.6)
  Top 0.3: v-90.63,19.05 -86.63,19.05 -86.33,18.75 -86.33,18.55 -85.63,17.85 R46.1
  Bottom 0.3: v-90.63,19.05 -90.83,18.85 -99.63,18.85 -105.43,13.05 -125.23,13.05 -131.93,19.75 -131.93,34.15 -128.93,37.15 -128.93,39.35 -127.23,39.35 IC6.10
N$168  (via drill 0.6)
  Top 0.3: v-114.23,21.75 -112.93,20.45 R30.1 | v-123.23,23.05 -124.43,24.25 -124.43,29.05 -127.13,31.75 IC6.13
  Bottom 0.3: v-114.23,21.75 -121.93,21.75 v-123.23,23.05
N$169  (via drill 0.6)
  Top 0.3: v-112.73,26.45 -112.73,23.05 -112.83,22.95 R45.1
  Bottom 0.3: v-112.73,26.45 -114.33,28.05 -128.13,28.05 -128.93,28.85 -128.93,34.25 -127.23,34.25 IC6.12
N$170  (via drill 0.6)
  Top 0.3: v-90.03,35.55 -90.03,25.05 -86.33,21.35 -86.33,21.15 -85.63,20.45 R31.1
  Bottom 0.3: v-90.03,35.55 -91.43,36.95 -117.23,36.95 -118.43,35.75 -126.03,35.75 -127.13,36.85 IC6.11
N$171  (via drill 0.6)
  Top 0.3: v-116.73,29.05 -116.73,22.65 -115.73,21.65 -115.73,20.65 -112.93,17.85 R33.1
  Bottom 0.3: v-116.73,29.05 -118.03,30.35 -126.13,30.35 -127.13,29.35 IC6.14
N$172  (via drill 0.6)
  Top 0.3: v-116.73,20.35 -116.73,19.15 -112.93,15.35 R47.1
  Bottom 0.3: v-116.73,20.35 -117.53,21.15 -129.33,21.15 -131.33,23.15 -131.33,26.65 -127.23,26.65 IC6.15
N$173
  Top 0.3: R32.1 -85.63,15.25 -86.33,14.55 -86.33,14.45 -89.13,11.65 -117.73,11.65 -117.73,37.25 -118.83,38.35 -125.43,38.35 -125.43,40.25 -127.13,41.95 IC6.9
N$174  (via drill 0.6)
  Top 0.3: v-109.43,34.55 -109.43,34.45 -111.63,34.45 -112.03,34.05 -112.03,33.95 -112.83,33.15 R48.1 | v-74.93,32.95 -71.33,29.35 IC7.13
  Bottom 0.3: v-109.43,34.55 -109.23,34.35 -84.33,34.35 -82.93,32.95 v-74.93,32.95
N$175  (via drill 0.6)
  Top 0.3: v-108.43,28.05 -108.43,36.95 -111.63,36.95 -112.03,36.55 -112.03,36.45 -112.83,35.65 R34.1
  Bottom 0.3: v-108.43,28.05 -107.13,26.75 -81.13,26.75 -80.03,25.65 -72.33,25.65 -71.33,26.65 IC7.12
N$176  (via drill 0.6)
  Top 0.3: v-83.63,35.05 -85.53,33.15 R49.1
  Bottom 0.3: v-83.63,35.05 -83.23,35.45 -69.93,35.45 -68.93,34.45 -68.93,24.25 -71.23,24.25 IC7.11
N$177  (via drill 0.6)
  Top 0.3: v-81.03,21.55 -83.23,23.75 -83.23,25.65 -85.53,27.95 R35.1
  Bottom 0.3: v-81.03,21.55 -80.03,20.55 -72.33,20.55 -71.33,21.55 IC7.10
N$178  (via drill 0.6)
  Top 0.3: v-75.43,19.55 -75.43,20.25 -81.13,20.25 -83.83,22.95 -83.83,23.75 -85.53,25.45 R50.1
  Bottom 0.3: v-75.43,19.55 -75.03,19.15 -71.33,19.15 IC7.9
N$179  (via drill 0.6)
  Top 0.3: v-112.03,28.95 -112.03,29.65 -112.83,30.45 R36.1
  Bottom 0.3: v-112.03,28.95 -111.73,29.25 -81.13,29.25 -80.03,28.15 -74.63,28.15 -72.13,30.65 -70.23,30.65 -69.53,31.35 -69.53,34.25 -71.23,34.25 IC7.15
N$180  (via drill 0.6)
  Top 0.3: v-83.63,30.55 -85.53,30.55 R51.1
  Bottom 0.3: v-83.63,30.55 -83.53,30.65 -72.93,30.65 -71.83,31.75 -71.33,31.75 IC7.14
N$181
  Top 0.3: R30.2 -110.93,20.35 -106.83,20.35 LED18.16
N$182
  Top 0.3: R45.2 -110.93,22.85 -106.83,22.85 LED18.15
N$183
  Top 0.3: R31.2 -87.53,20.35 -91.53,20.35 LED18.3
N$184
  Top 0.3: R32.2 -87.53,15.25 -91.53,15.25 LED18.1
N$185
  Top 0.3: R47.2 -110.93,15.25 -106.83,15.25 LED18.18
N$186
  Top 0.3: R33.2 -110.93,17.75 -106.83,17.75 LED18.17
N$187  (via drill 0.6)
  Top 0.3: v-109.43,33.15 -110.93,33.15 R48.2
  Bottom 0.3: v-109.43,33.15 -106.83,33.15 LED18.11
N$188  (via drill 0.6)
  Top 0.3: v-109.43,35.95 -109.43,35.65 -110.93,35.65 R34.2
  Bottom 0.3: v-109.43,35.95 -109.23,35.75 -106.83,35.75 LED18.10
N$189  (via drill 0.6)
  Top 0.3: v-89.03,33.05 -87.53,33.05 R49.2
  Bottom 0.3: v-89.03,33.05 -91.53,33.05 LED18.8
N$190  (via drill 0.6)
  Top 0.3: v-89.03,27.95 -87.53,27.95 R35.2
  Bottom 0.3: v-89.03,27.95 -91.53,27.95 LED18.6
N$191  (via drill 0.6)
  Top 0.3: v-89.03,25.45 R50.2
  Bottom 0.3: v-89.03,25.45 -89.13,25.35 LED18.5
N$192  (via drill 0.6)
  Top 0.3: v-109.43,30.55 -110.93,30.55 R36.2
  Bottom 0.3: v-109.43,30.55 -106.83,30.55 LED18.12
N$193  (via drill 0.6)
  Top 0.3: v-89.03,30.45 -87.53,30.45 R51.2
  Bottom 0.3: v-89.03,30.45 -91.53,30.45 LED18.7
N$194  (via drill 0.6)
  Top 0.3: v-120.73,22.75 -120.73,18.85 -122.03,17.55 IC2.1 | v-115.73,23.05 -115.73,42.45 -116.83,43.55 v-116.83,45.95
  Bottom 0.3: v-120.73,22.75 -120.43,23.05 v-115.73,23.05 | v-116.83,45.95 -116.23,46.55 -114.93,46.55 -108.13,53.35 JP14.16
N$195  (via drill 0.6)
  Top 0.3: v-122.83,15.25 -122.83,16.95 -123.33,17.45 IC2.2 | v-105.83,16.55 -105.63,16.75 -105.63,53.35 JP14.14
  Bottom 0.3: v-122.83,15.25 -121.53,16.55 v-105.83,16.55
N$196  (via drill 0.6)
  Top 0.3: IC2.3 -124.13,17.05 v-124.13,15.85 | v-104.63,19.15 -104.83,19.35 -104.83,51.55 -103.03,53.35 JP14.12
  Bottom 0.3: v-124.13,15.85 -121.23,18.75 -107.43,18.75 -107.03,19.15 v-104.63,19.15
N$197  (via drill 0.6)
  Top 0.3: v-121.73,24.15 -121.73,23.15 -125.43,19.45 -125.43,17.95 -125.83,17.55 IC2.4 | v-103.83,24.15 -100.53,27.45 -100.53,53.35 JP14.10
  Bottom 0.3: v-121.73,24.15 -120.43,25.45 -108.33,25.45 -107.03,24.15 v-103.83,24.15
N$198  (via drill 0.6)
  Top 0.3: v-126.63,15.85 -126.63,16.95 -127.13,17.45 IC2.5 | v-105.83,14.05 -98.03,21.85 -98.03,53.35 JP14.8
  Bottom 0.3: v-126.63,15.85 -124.83,14.05 v-105.83,14.05
N$199  (via drill 0.6)
  Top 0.3: v-127.93,19.25 -127.93,17.95 -128.33,17.55 IC2.6 | v-97.03,23.15 -95.43,24.75 -95.43,53.35 JP14.6
  Bottom 0.3: v-127.93,19.25 -127.83,19.35 -109.33,19.35 -107.03,21.65 -105.23,21.65 -103.73,23.15 v-97.03,23.15
N$200
  Top 0.3: IC2.7 -129.63,17.45 -129.23,17.05 -129.23,16.55 -123.73,11.05 -84.43,11.05 -84.43,16.15 -84.83,16.55 -93.33,16.55 -93.33,52.95 -92.93,53.35 JP14.4
N$201  (via drill 0.6)
  Top 0.3: v-129.33,41.95 -129.33,23.15 -130.43,22.05 -130.43,18.05 -130.93,17.55 IC2.8
  Bottom 0.3: v-129.33,41.95 -126.33,44.95 -98.73,44.95 -90.33,53.35 JP14.2
N$213
  Top 0.3: R58.1 -137.22,94 -129.17,102.05 -119.72,102.05 -119.72,102.75 IC13.6
N$214
  Top 0.3: R62.1 -129.52,94 -123.22,100.3 -119.72,100.3 IC13.7
N$215
  Top 0.3: R59.1 -121.82,93.65 -115.52,87.35 -115.52,87 -114.82,86.3 -112.02,86.3 -112.02,97.5 IC13.9
N$216
  Top 0.3: R63.1 -114.12,94 -113.77,94.35 -113.77,98.55 -112.02,100.3 IC13.10
N$217
  Top 0.3: R60.1 -109.92,96.8 -109.92,101 -111.67,102.75 IC13.11
N$218
  Top 0.3: R64.1 -99.42,94 -110.62,105.2 -111.67,105.2 IC13.12
N$219
  Top 0.3: R57.2 -152.62,91.55 -152.62,87.7 LED21.A
N$220
  Top 0.3: R61.2 -144.92,91.55 -144.92,87.7 LED25.A
N$221
  Top 0.3: R58.2 -137.22,91.55 -137.22,87.7 LED22.A
N$222
  Top 0.3: R62.2 -129.52,91.55 -129.52,87.7 LED26.A
N$223
  Top 0.3: R59.2 -121.82,91.55 -121.82,87.7 LED23.A
N$224
  Top 0.3: R63.2 -114.47,91.55 -114.47,87.7 LED27.A
N$225
  Top 0.3: R60.2 -106.77,91.55 -106.77,87.7 LED24.A
N$226
  Top 0.3: R64.2 -99.07,91.55 -99.07,87.7 LED28.A
N$227
  Bottom 0.3: ADU_DAU.11 -131.27,127.25 -134.42,130.4 -138.62,130.4 -141.77,127.25 -142.12,127.25 OSC.1
N$228
  Top 0.3: Q2.2 -146.32,110.8 -152.27,110.8 IC14.1
N$229
  Top 0.3: PTC.1 EEPROM.7
N$230
  Top 0.3: U$1.3 -154.37,126.9 -154.02,126.55 -154.02,125.85 -151.57,123.4 -147.72,123.4 OS.1
N$231
  Bottom 0.3: ADU_DAU.15 -120.77,126.9 -117.97,124.1 -115.52,124.1 -112.72,126.9 -112.02,126.9 AOUT.1
N$232
  Top 0.3: Q2.1 -146.32,115.35 -150.52,115.35 -150.52,115 -152.27,113.25 IC14.2
N$233
  Top 0.3: INT.1 IC13.13
N$234
  Top 0.3: IC12.13 -90.32,127.25 -85.42,127.25 INT4.1
N$235
  Top 0.3: IC14.7 -160.32,113.25 -165.22,113.25 INT5.1
N$236  (via drill 0.6)
  Top 0.3: v-124.27,138.1 -128.82,142.65 -128.82,144.4 -130.22,145.8 -157.52,145.8 -157.52,143.7 R65.S
  Bottom 0.3: v-124.27,138.1 -121.12,134.95 ADU_DAU.2
N$237
  Top 0.3: ADU_DAU.3 -123.57,134.6 -125.32,132.85 -129.52,132.85 -129.52,144.05 -130.57,145.1 -135.82,145.1 -135.82,143.7 R66.S
N$238
  Top 0.3: ADU_DAU.1 -117.97,134.95 -106.07,134.95 -106.07,137.4 -98.37,145.1 -93.12,145.1 -93.12,143.7 R68.S
N$239
  Top 0.3: ADU_DAU.4 -125.67,134.95 -121.12,139.5 -121.12,144.05 -120.07,145.1 -114.47,145.1 -114.47,143.7 R67.S
RA0
  Top 0.3: U1.2 -28.13,49.52 -39.43,38.22 -39.43,34.42 JP4.6
RA1
  Top 0.3: U1.3 -25.63,49.52 -36.93,38.22 -36.93,34.42 JP4.5
RA2
  Top 0.3: U1.4 -23.03,49.52 -34.43,38.12 -34.43,34.42 JP4.4
RA3
  Top 0.3: U1.5 -31.83,38.22 -31.83,34.42 JP4.3
RA4
  Top 0.3: U1.6 -17.93,49.52 -29.33,38.12 -29.33,34.42 JP4.2
RA5
  Top 0.3: U1.7 -15.43,49.52 -26.73,38.22 -26.73,34.42 JP4.1
RB0
  Top 0.3: JP9.1 -11.63,107.92 -11.63,105.02 -12.53,104.12 INT1.2 -12.53,104.02 -12.53,94.22 INT1.1 -12.53,94.02 R71.2 -12.53,88.92 -12.83,88.62 -12.83,85.22 JP6.8 -12.83,85.02 -12.83,64.82 U1.33
RB1
  Top 0.3: JP12.1 -17.93,105.02 -17.03,104.12 INT3.1 -16.93,104.02 -16.93,94.22 INT3.2 -17.03,94.02 -17.03,92.02 -18.03,91.02 | -18.03,91.02 -19.13,89.92 R70.2 | U1.34 -15.43,64.82 -15.43,85.12 JP6.7 -15.43,85.22 -15.43,88.42 -18.03,91.02
RB2
  Top 0.3: INT2.1 -27.03,104.02 -27.03,94.12 INT2.2 -26.93,94.02 -26.83,93.92 -26.83,63.02 | -26.83,63.02 -17.93,63.02 U1.35 JP11.1 JP6.6 | -26.83,63.02 -28.93,63.02 -34.73,57.22 R69.2
RB3
  Top 0.3: U1.36 -20.43,64.82 -20.43,85.12 JP6.5
RB4
  Top 0.3: U1.37 -23.03,64.82 -23.03,85.12 JP6.4
RB5  (via drill 0.6)
  Top 0.3: v-31.63,81.42 -33.43,81.42 R10.1
  Bottom 0.3: JP6.3 -25.63,85.12 -27.63,83.12 -29.93,83.12 v-31.63,81.42 -31.63,66.62 | -31.63,66.62 -40.23,66.62 -40.73,66.12 ICSP.6 | -31.63,66.62 -27.43,66.62 -25.63,64.82 U1.38
RB6
  Top 0.3: R5.1 -28.03,68.92 -28.03,64.82 U1.39
  Bottom 0.3: ICSP.5 -40.73,63.52 -40.23,63.02 -29.93,63.02 -28.13,64.82 U1.39
RB7
  Top 0.3: U1.40 R8.1
  Bottom 0.3: U1.40 -42.73,64.82 -42.73,62.92 -40.83,61.02 ICSP.4
RC0
  Top 0.3: U1.15 4.47,49.12 4.47,37.72 1.17,34.42 JP8.8
RC1
  Top 0.3: U1.16 7.47,49.52 5.07,47.12 5.07,35.82 3.67,34.42 JP8.7
RC2
  Top 0.3: U1.17 9.97,49.52 6.27,45.82 6.27,34.42 JP8.6
RC3
  Top 0.3: U1.18 12.47,49.52 12.47,33.12 11.67,32.32 8.77,32.32 8.77,34.32 JP8.5
RC4
  Top 0.3: U1.23 12.47,64.82 11.37,63.72 11.37,34.42 JP8.4
RC5
  Bottom 0.3: U1.24 10.07,64.82 10.07,63.02 13.77,59.32 13.77,34.42 JP8.3
RC6
  Bottom 0.3: U1.25 7.47,63.12 11.47,59.12 11.47,36.32 11.77,36.32 12.57,35.52 12.57,32.32 14.27,32.32 16.27,34.32 JP8.2
RC7
  Bottom 0.3: U1.26 4.97,64.82 8.87,60.92 8.87,36.32 9.17,36.32 10.07,35.42 10.07,31.72 16.27,31.72 18.87,34.32 JP8.1
RD0
  Top 0.3: JP7.8 13.67,84.02 13.67,51.02 15.07,49.62 U1.19
RD1
  Bottom 0.3: U1.20 17.57,49.62 17.57,63.02 17.27,63.02 16.17,64.12 16.17,83.12 12.07,83.12 10.07,85.12 JP7.7
RD2
  Bottom 0.3: U1.21 17.57,64.82 17.57,83.12 17.07,83.12 13.07,87.12 9.37,87.12 7.47,85.22 JP7.6
RD3
  Bottom 0.3: U1.22 15.07,64.82 4.97,74.92 4.97,85.12 JP7.5
RD4
  Top 0.3: U1.27 2.37,64.82 2.37,85.12 JP7.4
RD5
  Top 0.3: U1.28 -0.13,64.82 -0.13,85.12 JP7.3
RD6
  Top 0.3: U1.29 -2.73,64.82 -2.73,85.12 JP7.2
RD7
  Top 0.3: JP7.1 U1.30
RE0
  Top 0.3: TP1.TP -20.43,34.42 -19.23,35.62 -19.23,43.22 JP1.3 -19.13,43.32 -12.93,49.52 U1.8
RE1
  Top 0.3: TP2.TP -16.63,34.42 -16.63,43.22 JP1.2 -16.53,43.32 -10.33,49.52 U1.9
RE2
  Top 0.3: JP2.2 -9.13,34.32 -12.83,34.32 TP3.TP -14.03,35.52 -14.03,43.12 JP1.1 U1.10
RESET
  Top 0.3: S2.1 -40.83,79.02 -40.83,73.72 C4.+ | D2.A -52.23,49.62 -52.23,69.82 D1.A -52.13,69.92 -52.13,70.92 -49.43,73.62 R1.1 -49.43,73.82 -49.43,77.62 -50.83,79.02 S2.2
  Bottom 0.3: C4.+ -40.83,73.62 -43.43,71.02 -51.03,71.02 -52.13,69.92 D1.A
RESETSPI  (via drill 0.6)
  Top 0.3: v-147.23,14.55 -147.23,16.05 -147.43,16.25 IC3.18 | v-136.33,10.65 -134.83,9.15 -134.83,8.05 IC2.18 | v-156.13,4.05 -156.13,-8.55 -161.43,-13.85 SPI_INPUT.4
  Bottom 0.3: -146.43,13.75 -143.33,10.65 v-136.33,10.65 | -146.43,13.75 v-147.23,14.55 | -146.43,13.75 v-156.13,4.05
RX
  Bottom 0.3: 39.26,18.88 JP17.2 39.36,18.78 43.06,15.08 43.06,-15.22 44.36,-16.52 44.36,-19.22 44.96,-19.82 47.96,-19.82 47.96,-18.02 JP16.3
SCK  (via drill 0.6)
  Top 0.3: IC2.12 -136.13,17.55 -136.13,18.85 -139.03,18.85 -139.33,18.55 -139.33,17.95 -145.73,11.55 -145.73,7.15 -146.13,6.75 IC3.12 -146.33,6.65 -146.33,1.85 v-148.03,0.15
  Bottom 0.3: v-148.03,0.15 -155.03,0.15 -169.03,-13.85 SPI_INPUT.7
SCL  (via drill 0.6)
  Top 0.3: IC13.14 -111.67,110.8 -95.57,110.8 -95.57,124.1 -90.32,129.35 IC12.14 | -130.92,117.1 -130.92,124.45 -133.37,126.9 ADU_DAU.10 | -130.92,117.1 -130.92,108.7 -132.67,108.7 -133.37,109.4 -133.37,112.55 -135.47,112.55 -137.22,110.8 EEPROM.6 | -156.12,120.6 -156.12,119.55 -159.97,115.7 IC14.6 -160.32,115.7 -162.07,117.45 -162.07,121.65 -168.72,128.3 I2C-INPUT.2 | -156.12,120.6 -156.12,126.55 -155.77,126.9 U$1.2 | -156.12,120.6 v-148.77,120.6 | -130.92,117.1 v-119.02,117.1 | v-163.03,114.93 -163.03,115.53 -165.53,115.53 R73.2
  Bottom 0.3: v-148.77,120.6 -147.02,120.6 -141.77,115.35 -137.57,115.35 -137.57,110.8 EEPROM.6 | v-119.02,117.1 -118.32,117.1 -112.02,110.8 IC13.14 | v-163.03,114.93 -162.43,115.53 -160.23,115.53 IC14.6
SDA
  Top 0.3: -159.97,122 -159.97,118.5 IC14.5 | -159.97,122 -159.97,124.1 -157.17,126.9 U$1.1 | -159.97,122 -168.72,130.75 I2C-INPUT.3 -169.07,130.75 -171.17,128.65 -171.17,117.1 -163.47,109.4 -162.63,109.4 | EEPROM.5 -139.67,110.8 -136.17,114.3 -136.17,126.9 ADU_DAU.9 | IC12.15 -90.32,133.2 -99.07,133.2 -99.77,132.5 -99.77,125.15 -111.67,113.25 IC13.15 -112.02,112.9 -113.77,112.9 -114.47,112.2 -114.47,109.4 -120.42,109.4 -124.97,104.85 -124.97,104.15 -135.12,104.15 -136.17,105.2 -136.17,106.95 -139.67,110.45 EEPROM.5 | -162.63,109.4 -140.02,109.4 -140.02,110.45 EEPROM.5 | -162.63,109.4 -162.63,109.03 R72.2
SI  (via drill 0.6)
  Top 0.3: IC2.13 -137.33,17.45 -137.33,16.95 -144.43,9.85 -144.43,7.25 -144.93,6.75 IC3.13 -145.03,6.65 -145.03,0.15 v-148.23,-3.05
  Bottom 0.3: v-148.23,-3.05 -155.63,-3.05 -166.43,-13.85 SPI_INPUT.6
SO  (via drill 0.6)
  Top 0.3: v-143.03,-12.45 -143.03,-4.08 | -143.03,-4.08 -143.03,6.05 -143.63,6.65 IC3.14 | -143.03,-4.08 -148.73,-4.08 -151.23,-6.58 R74.2
  Bottom 0.3: v-143.03,-12.45 -143.33,-12.75 -150.43,-12.75 -152.63,-14.95 -152.63,-15.85 -162.03,-15.85 -163.93,-13.95 SPI_INPUT.5
SPI_A
  Top 0.3: IC3.1 -160.23,6.75 -165.83,12.35 -165.83,17.15 -167.73,19.05 KEYBOARD_INPUT.1
SPI_B  (via drill 0.6)
  Top 0.3: v-159.43,9.85 -159.43,7.25 -158.93,6.75 IC3.2
  Bottom 0.3: v-159.43,9.85 -166.13,16.55 -167.73,16.55 KEYBOARD_INPUT.2
SPI_C
  Top 0.3: IC3.3 -157.63,6.75 -158.13,7.25 -158.13,11.85 -166.63,20.35 -169.73,20.35 -169.73,15.95 -167.83,14.05 KEYBOARD_INPUT.3
SPI_D
  Top 0.3: IC3.4 -156.43,6.65 -156.83,6.25 -156.83,5.75 -157.13,5.45 -165.83,5.45 -165.83,9.55 -167.73,11.45 KEYBOARD_INPUT.4
SPI_E  (via drill 0.6)
  Top 0.3: v-155.63,8.35 -155.63,7.25 -155.13,6.75 IC3.5
  Bottom 0.3: v-155.63,8.35 -156.13,8.85 -167.73,8.85 KEYBOARD_INPUT.5
SPI_F
  Top 0.3: IC3.6 -153.83,6.65 -154.33,6.15 -154.33,5.65 -154.93,5.05 -156.73,5.05 -156.93,4.85 -166.33,4.85 -166.33,4.95 -167.73,6.35 KEYBOARD_INPUT.6
SPI_G  (via drill 0.6)
  Top 0.3: v-154.53,2.65 -152.53,4.65 -152.53,6.65 IC3.7
  Bottom 0.3: v-154.53,2.65 -154.93,3.05 -166.93,3.05 -167.73,3.85 KEYBOARD_INPUT.7
SPI_H  (via drill 0.6)
  Top 0.3: IC3.8 -151.73,6.25 -151.73,4.05 v-153.13,2.65
  Bottom 0.3: v-153.13,2.65 -154.43,1.35 -167.73,1.35 KEYBOARD_INPUT.8
SPIGND
  pour Bottom (isolate 0.406): -174.14,-21.54 -174.14,64.82 -172.87,66.09 -63.65,66.09 -62.38,64.82 -62.38,-21.54 -63.65,-22.81 -172.87,-22.81
TX
  Bottom 0.3: 47.91,18.83 JP18.2 47.96,18.88 45.86,16.78 45.86,-17.72 JP16.2
VCC  (via drill 0.6)
  Top 0.8: LED16.A -52.23,148.62 -52.23,141.32 LED15.A -52.23,133.72 LED14.A -52.23,133.32 -52.23,126.12 LED13.A -52.23,125.72 -52.23,118.52 LED12.A -52.23,118.12 -52.23,110.92 LED11.A -52.23,110.52 -52.23,103.22 LED10.A -52.23,95.32 LED9.A -52.33,94.92 -52.33,94.52 -54.23,92.62 -54.23,83.52 -51.73,81.02 -48.03,81.02 -47.73,80.82 -47.73,74.02 R1.2 -47.43,73.62 -44.63,70.82 -44.63,69.92 D1.C -44.33,69.62 -44.33,56.12 | LED1.A -38.23,151.22 -30.63,151.22 LED2.A -30.33,151.22 -23.03,151.22 LED3.A -22.63,151.22 -15.43,151.22 LED4.A -15.03,151.22 -7.83,151.22 LED5.A -7.43,151.22 -0.23,151.22 LED6.A 0.17,151.22 7.47,151.22 LED7.A 7.77,151.22 15.07,151.22 LED8.A | 16.42,6.57 17.77,5.22 18.87,5.22 IR1.VS | 16.42,6.57 14.87,8.12 14.87,16.82 11.37,20.32 JP3.1 10.87,20.42 0.27,31.02 -2.73,31.02 -2.73,46.92 -5.03,49.22 U1.11 -5.23,49.62 -9.03,53.42 -9.03,55.72 | C7.1 -2.63,-10.08 11.27,-10.08 C8.+ 11.47,-9.78 11.47,1.62 16.42,6.57 | -36.83,55.92 -36.83,57.02 -36.73,57.12 R69.1 | -36.83,55.92 -37.73,55.02 -40.73,55.02 -40.73,55.92 ICSP.2 -41.13,56.12 -44.33,56.12 | C1.+ -53.43,33.12 -52.73,33.82 -52.73,41.92 C9.+ -52.53,42.32 -50.23,44.62 -50.23,50.12 -44.53,55.82 -44.33,56.12 | -9.03,55.72 -9.03,63.62 -10.23,64.82 U1.32 -10.53,65.12 -11.43,66.02 -11.43,87.12 v-11.73,87.32 -10.63,88.42 R71.1 -10.53,89.32 -10.53,90.22 TP5.TP -7.43,90.02 12.77,90.02 17.57,85.22 JP19.1 | v-16.43,87.92 -19.13,87.92 R70.1 | -9.03,55.72 -36.53,55.72 -36.83,55.92
  Bottom 0.8: LED16.A -52.13,148.72 -49.73,151.12 -38.33,151.12 LED1.A | IC1.3 -20.43,-15.18 -15.43,-10.18 -2.73,-10.18 C7.1 | C10.2 -48.43,22.92 -53.43,22.92 +5V.1 -53.43,23.32 -53.43,33.02 C1.+ | v-16.43,87.92 -15.83,87.32 v-11.73,87.32
VCC_COM  (via drill 0.6)
  Top 0.3: IC11.16 48.26,49.63 48.26,53.13 C14.1 | LED20.A 65.66,7.48 59.36,1.18 47.86,1.18 47.86,2.38 IC10.4 | 44.56,-1.22 44.56,-0.32 35.46,-0.32 R54.1 | 44.56,-1.22 44.56,-4.82 IC10.20 | v49.96,-1.22 44.56,-1.22
  Bottom 0.3: 43.01,44.38 47.91,49.28 IC11.16 48.26,49.28 59.36,49.28 | 65.76,49.28 59.36,49.28 | 58.56,-9.82 65.66,-2.72 65.66,7.48 LED20.A 65.66,7.78 65.66,14.08 59.66,20.08 LED19.A 59.36,20.38 59.36,49.28 | 58.56,-9.82 JP16.4 | 58.56,-9.82 v49.96,-1.22
VCCI2C  (via drill 0.6)
  Top 0.3: -97.67,142.3 -90.32,134.95 IC12.16 | -97.67,142.3 -97.67,143.35 R68.E | IC13.3 -119.37,110.8 -119.37,112.9 IC13.2 -119.37,113.25 -119.37,115.35 IC13.1 -119.37,115.7 -117.97,115.7 | -117.97,115.7 -112.02,115.7 IC13.16 | -119.37,129 -118.32,129 -118.32,127.25 ADU_DAU.16 -117.97,126.9 -117.97,115.7 | -119.37,129 -121.47,129 -123.22,127.25 ADU_DAU.14 -123.57,127.25 -125.32,129 -134.77,129 | -119.37,129 -119.37,132.85 | -119.37,132.85 -119.37,143.35 R67.E | -97.67,142.3 -107.12,132.85 -119.37,132.85 | -156.47,114.3 -154.37,116.4 -152.62,116.4 -152.62,115.7 IC14.3 -152.27,115.7 -145.97,122 -145.97,132.15 | -156.47,114.3 -159.97,110.8 IC14.8 | -163.24,120.02 -162.77,119.55 -162.77,116.05 -161.02,114.3 -156.47,114.3 | -163.24,120.02 -168.72,125.5 I2C-INPUT.1 | U$1.8 -156.82,132.15 -155.77,132.15 U$1.7 -155.77,132.5 -155.42,132.85 -155.42,133.2 -152.97,135.65 | -152.97,135.65 -152.97,143.35 R65.A | -152.97,135.65 -152.97,132.5 U$1.5 -152.97,132.15 -145.97,132.15 | EEPROM.8 -132.32,110.8 -132.32,115.7 EEPROM.2 -134.77,129 | R66.A -131.27,143.35 -131.27,137.05 -133.37,134.95 ADU_DAU.7 -133.72,134.6 -134.77,133.55 -134.77,132.15 | -134.77,132.15 -134.77,129 | -134.77,132.15 -145.97,132.15 | v-161.03,108.43 -161.03,107.13 -162.63,107.13 R72.1 | -163.24,120.02 -166.63,116.63 -166.63,116.43 -167.43,115.63 R73.1
  Bottom 0.3: v-161.03,108.43 -160.23,109.23 -160.23,110.53 IC14.8
VCCSPI  (via drill 0.6)
  Top 0.3: IC4.3 -71.23,-8.75 -71.23,-6.35 IC4.4 -71.23,-6.25 -71.23,-3.85 IC4.5 -71.23,-3.65 -69.53,-1.95 -69.53,15.15 -77.13,22.75 -77.13,25.05 -78.73,26.65 IC7.5 -78.83,26.75 -78.83,29.25 IC7.4 -78.83,29.35 -78.83,31.75 IC7.3 -78.73,31.85 -77.13,33.45 -77.13,33.95 -74.23,33.95 -71.33,36.85 IC7.16 | IC5.5 -127.13,-8.75 -127.13,-6.35 IC5.4 -127.13,-6.15 -127.13,-3.85 IC5.3 | v-150.03,4.05 -150.03,6.65 IC3.9 | v-146.03,-6.15 -149.84,-9.96 | -149.84,-9.96 -153.73,-13.85 SPI_INPUT.1 | IC6.5 IC6.4 IC6.3 -119.63,29.15 -123.23,25.55 v-123.23,24.45 | IC2.15 -138.53,7.95 -137.33,7.95 IC2.16 | IC2.17 -136.13,7.95 -137.23,7.95 IC2.16 | -135.43,12.95 -137.33,11.05 -137.33,8.05 IC2.16 | -135.43,12.95 -132.73,15.65 -132.73,16.95 -132.23,17.45 IC2.9 -132.23,21.65 v-130.33,23.55 -133.63,26.85 -133.63,48.25 IC9.1 -133.53,48.35 -133.53,55.85 IC9.16 | IC8.1 -160.13,35.65 -160.13,43.15 IC8.16 | IC5.16 -119.53,1.35 -121.33,3.15 -121.33,9.05 -122.73,10.45 -135.33,10.45 -135.33,12.85 -135.43,12.95 | -149.84,-9.96 -151.23,-8.58 R74.1
  Bottom 0.3: IC4.16 -78.83,-13.85 -78.23,-13.25 -75.73,-13.25 -71.33,-8.85 IC4.3 | -142.93,-3.05 -142.23,-3.75 -127.23,-3.75 IC5.3 -127.03,-3.75 -124.53,-3.75 -119.53,1.25 IC5.16 | -142.93,-3.05 v-150.03,4.05 | -142.93,-3.05 v-146.03,-6.15 | v-130.33,23.55 -127.83,23.55 -127.23,24.15 IC6.16 -127.03,24.25 -123.43,24.25 v-123.23,24.45 | -140.73,44.85 -137.33,48.25 -133.53,48.25 IC9.1 | -140.73,44.85 -142.33,43.25 IC8.9 | IC9.9 -115.73,55.85 -117.43,54.15 -131.73,54.15 -133.43,55.85 IC9.16 | IC8.16 -160.13,43.25 -158.43,44.95 -140.83,44.95 -140.73,44.85 | IC7.3 -78.93,31.85 -119.53,31.85 IC6.4

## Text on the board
Top: Main Board | v1.1 | interrupts | reset | Pic 18 | Denys Maiier
Bottom: I²C / v1.1 | SPI / v1.1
